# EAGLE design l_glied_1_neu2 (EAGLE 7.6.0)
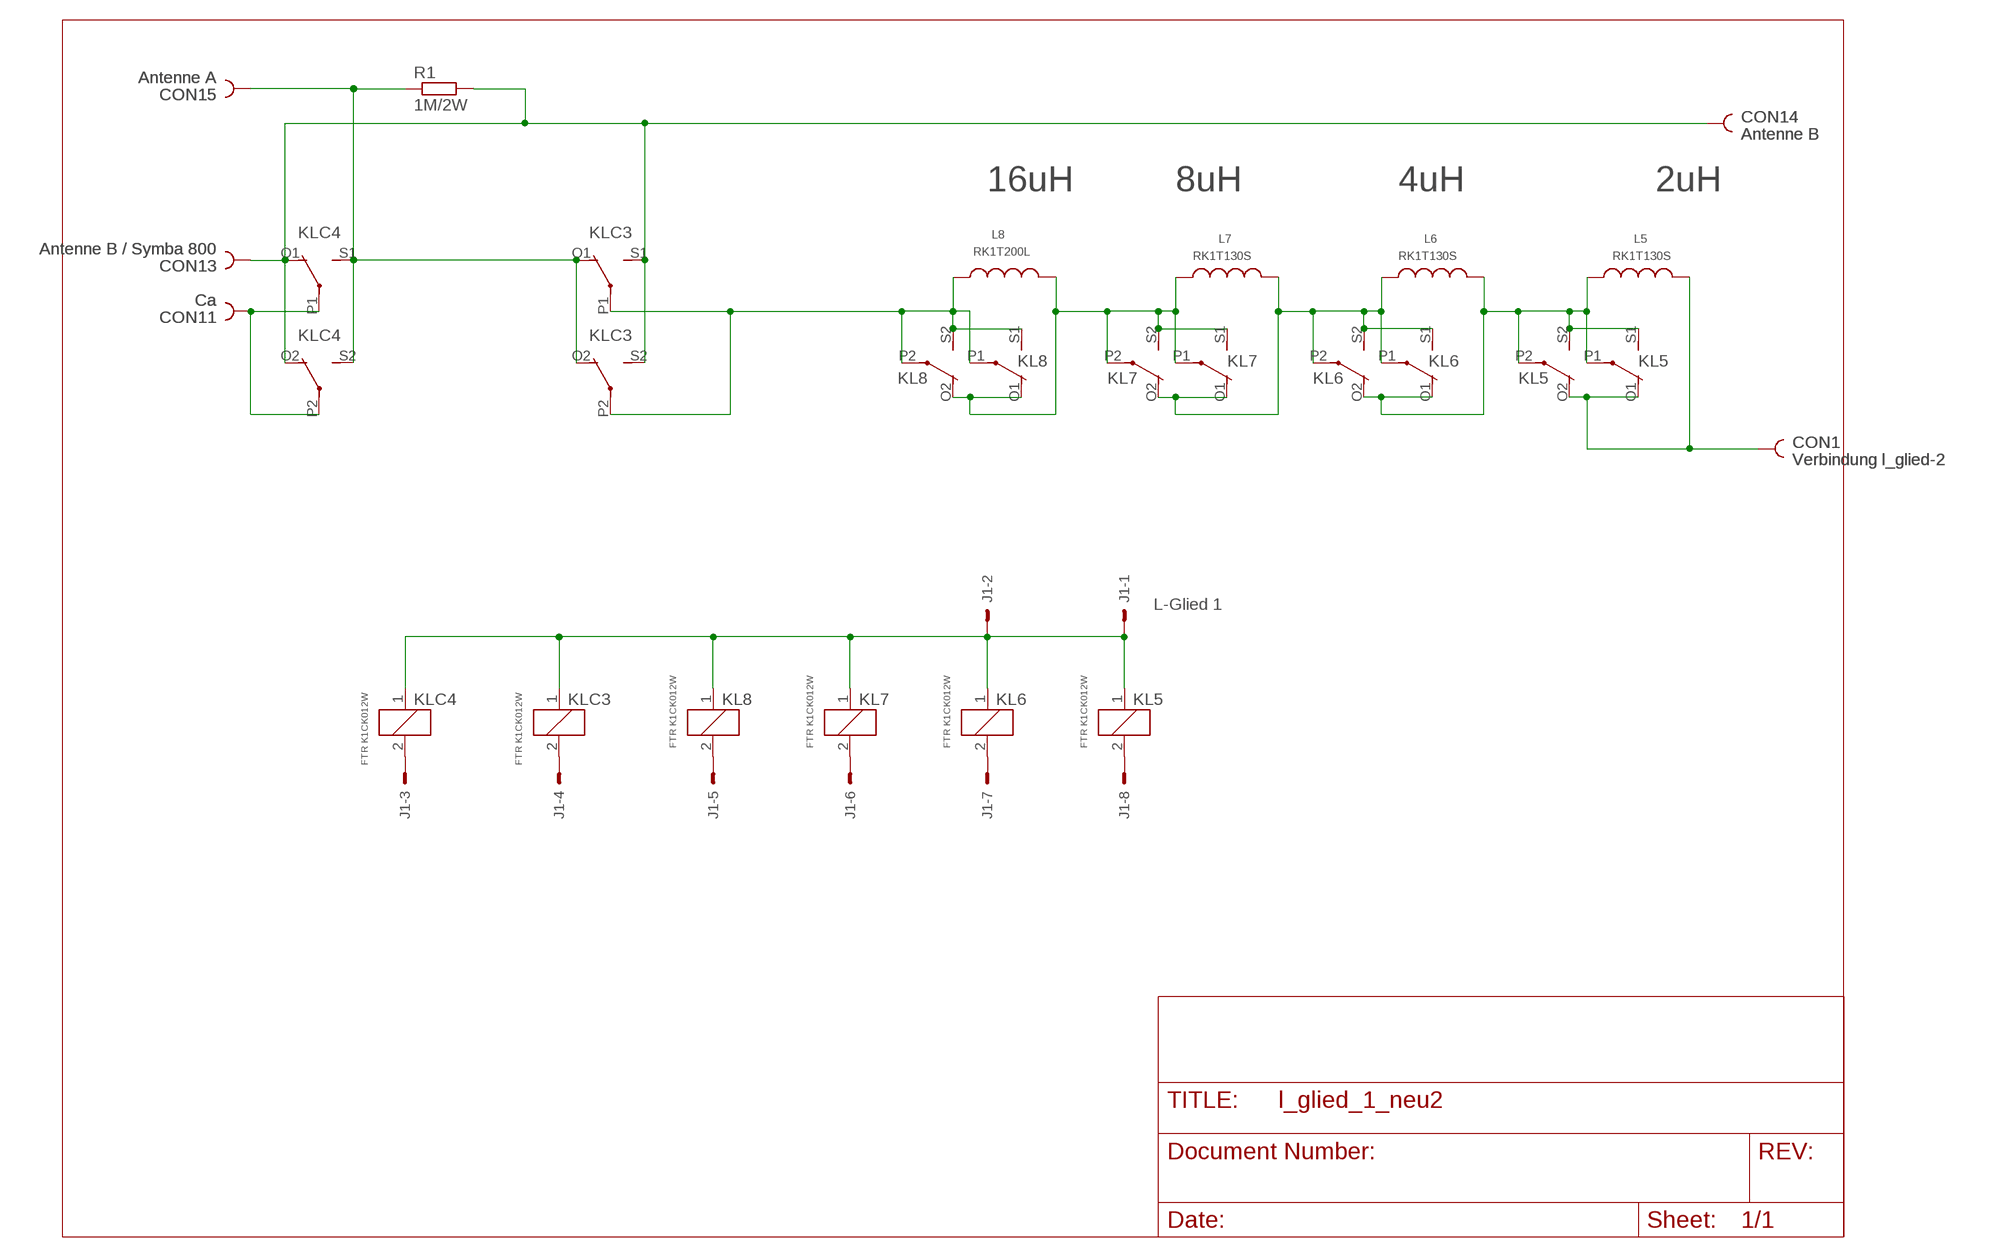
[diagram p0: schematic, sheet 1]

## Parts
CON1  Verbindung l_glied-2  PIN2_53MM  [HOLE3]
CON11  Ca  PIN2_53MM  [HOLE3]
CON13  Antenne B / Symba 800  PIN2_53MM  [HOLE3]
CON14  Antenne B  PIN2_53MM  [HOLE3]
CON15  Antenne A  PIN2_53MM  [HOLE3]
J1  L-Glied 1  22-27-2081-08  [6410-08]
KL5  FTR K1CK012W  4052  [F4052]
KL6  FTR K1CK012W  4052  [F4052]
KL7  FTR K1CK012W  4052  [F4052]
KL8  FTR K1CK012W  4052  [F4052]
KLC3  FTR K1CK012W  4052  [F4052]
KLC4  FTR K1CK012W  4052  [F4052]
L5  RK1T130S  [T130S]
L6  RK1T130S  [T130S]
L7  RK1T130S  [T130S]
L8  RK1T200L  [T200L]
R1  1M/2W  R-EU_R2512  [R2512]

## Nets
N$1: KL7.P1(2:P) KL7.P2(3:P) KL7.S1(2:S) KL7.S2(3:S) KL8.O1(2:O) KL8.O2(3:O) L7.1 L8.2
N$2: J1.5 KL8.2
N$3: KL5.P1(2:P) KL5.P2(3:P) KL5.S1(2:S) KL5.S2(3:S) KL6.O1(2:O) KL6.O2(3:O) L5.1 L6.2
N$4: J1.6 KL7.2
N$5: J1.7 KL6.2
N$6: J1.4 KLC3.2
N$7: J1.8 KL5.2
N$8: CON13.1 CON14.1 KLC3.S1(2:S) KLC3.S2(3:S) KLC4.O1(2:O) KLC4.O2(3:O) R1.2
N$9: CON15.1 KLC3.O1(2:O) KLC3.O2(3:O) KLC4.S1(2:S) KLC4.S2(3:S) R1.1
N$11: J1.3 KLC4.2
N$15: CON11.1 KLC4.P1(2:P) KLC4.P2(3:P)
N$16: KL8.P1(2:P) KL8.P2(3:P) KL8.S1(2:S) KL8.S2(3:S) KLC3.P1(2:P) KLC3.P2(3:P) L8.1
N$18: J1.1 J1.2 KL5.1 KL6.1 KL7.1 KL8.1 KLC3.1 KLC4.1
N$37: KL6.P1(2:P) KL6.P2(3:P) KL6.S1(2:S) KL6.S2(3:S) KL7.O1(2:O) KL7.O2(3:O) L6.1 L7.2
N$39: CON1.1 KL5.O1(2:O) KL5.O2(3:O) L5.2

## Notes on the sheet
- 16uH | 8uH | 4uH | 2uH

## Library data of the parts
CON1 CON11 CON13-CON15 = lindenau:PIN2_5
J1 = con-molex:22-?-08: CONNECTOR wire to board 2.54 mm (.1 inch) pitch header; OC_FARNELL: unknown; OC_NEWARK: unknown
KL5-KL8 KLC3 KLC4 = relay:4052: RELAY 2 x switch, Finder; OC_FARNELL: unknown; OC_NEWARK: unknown
L5-L8 = lindenau:RK1
R1 = rcl:R-EU_: RESISTOR, European symbol

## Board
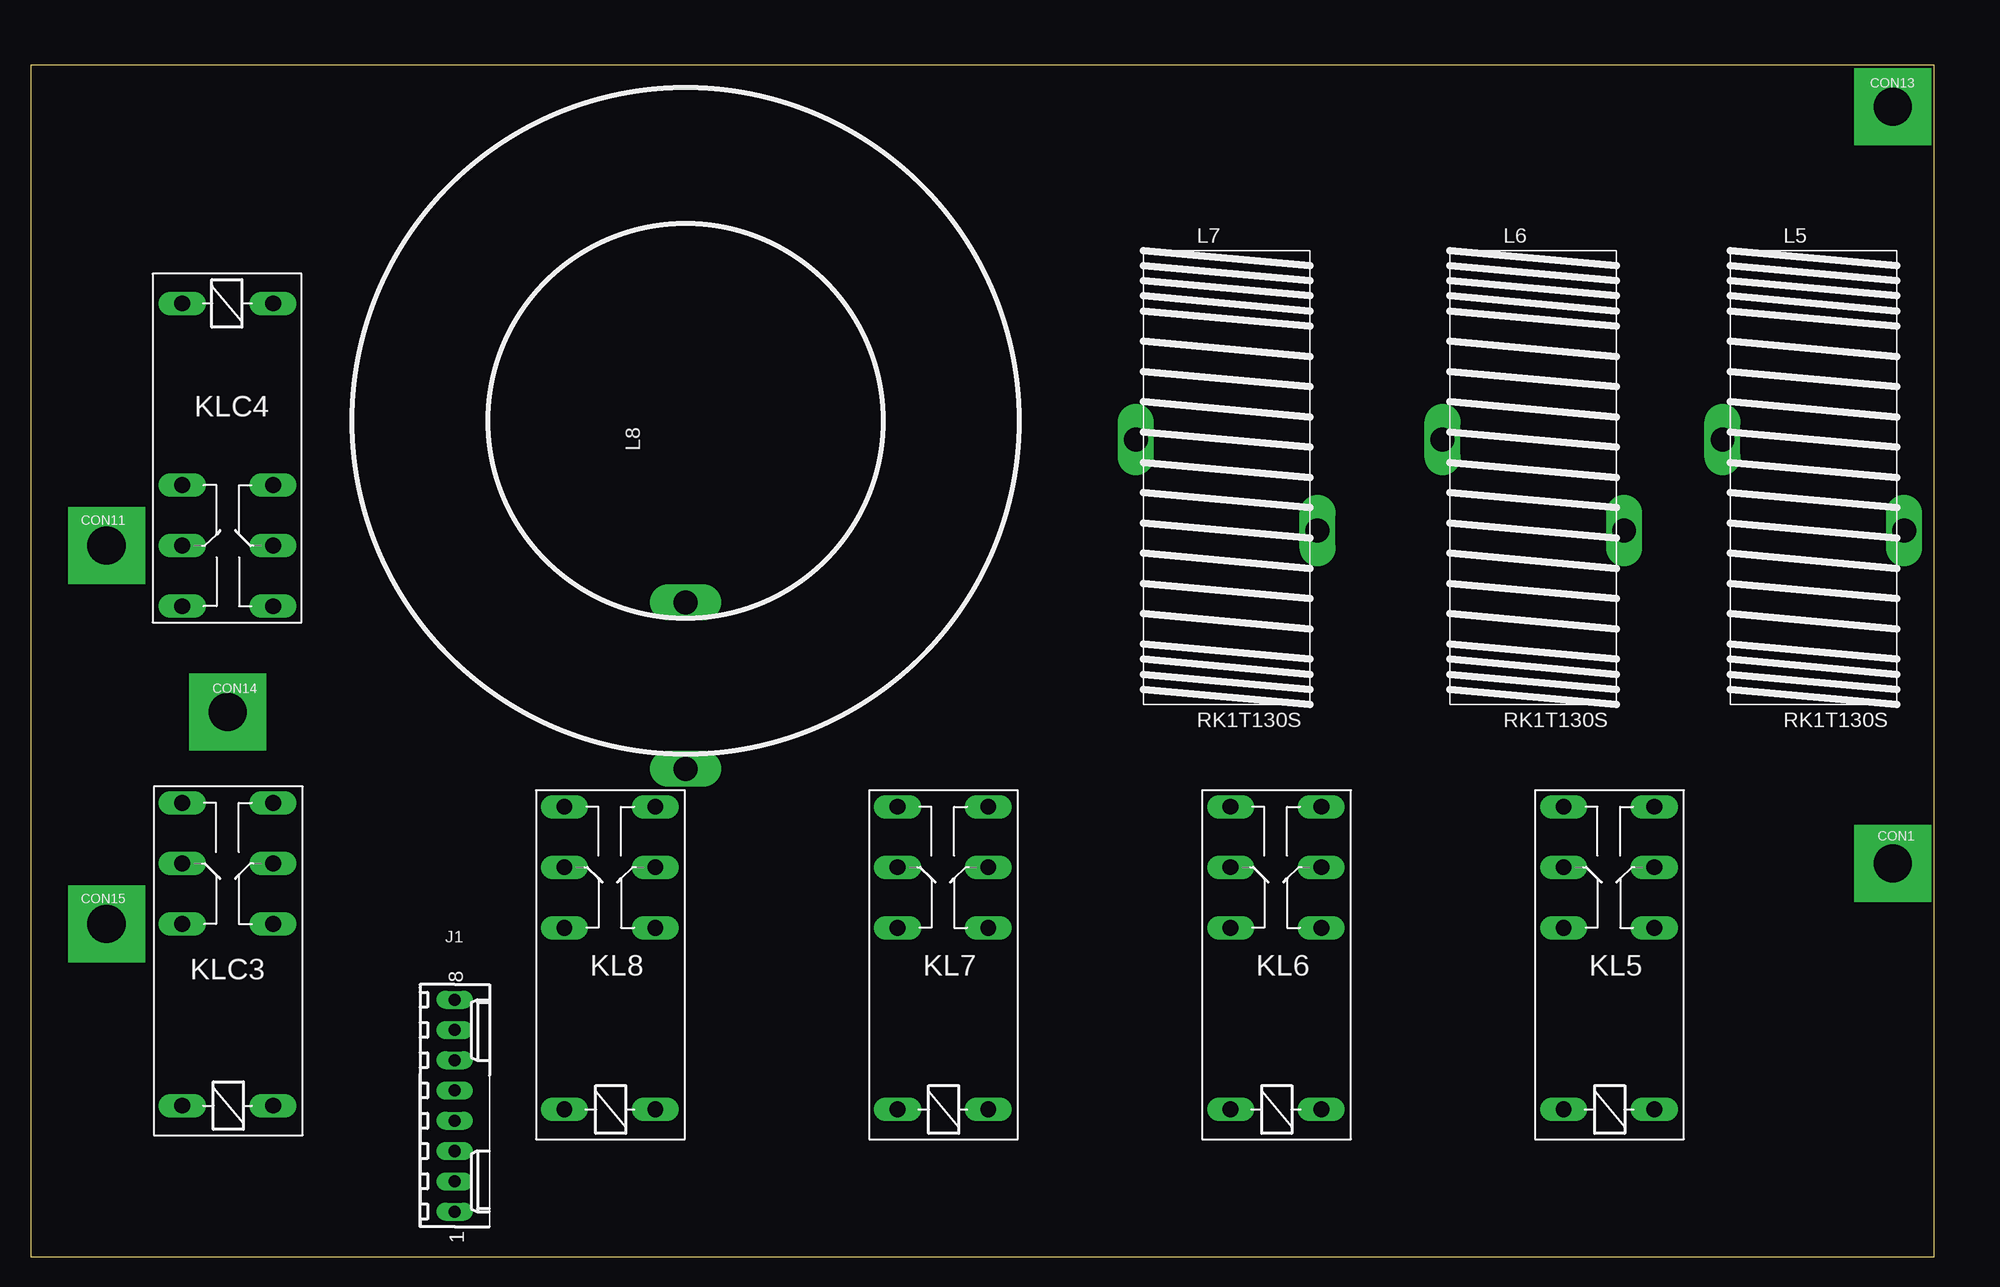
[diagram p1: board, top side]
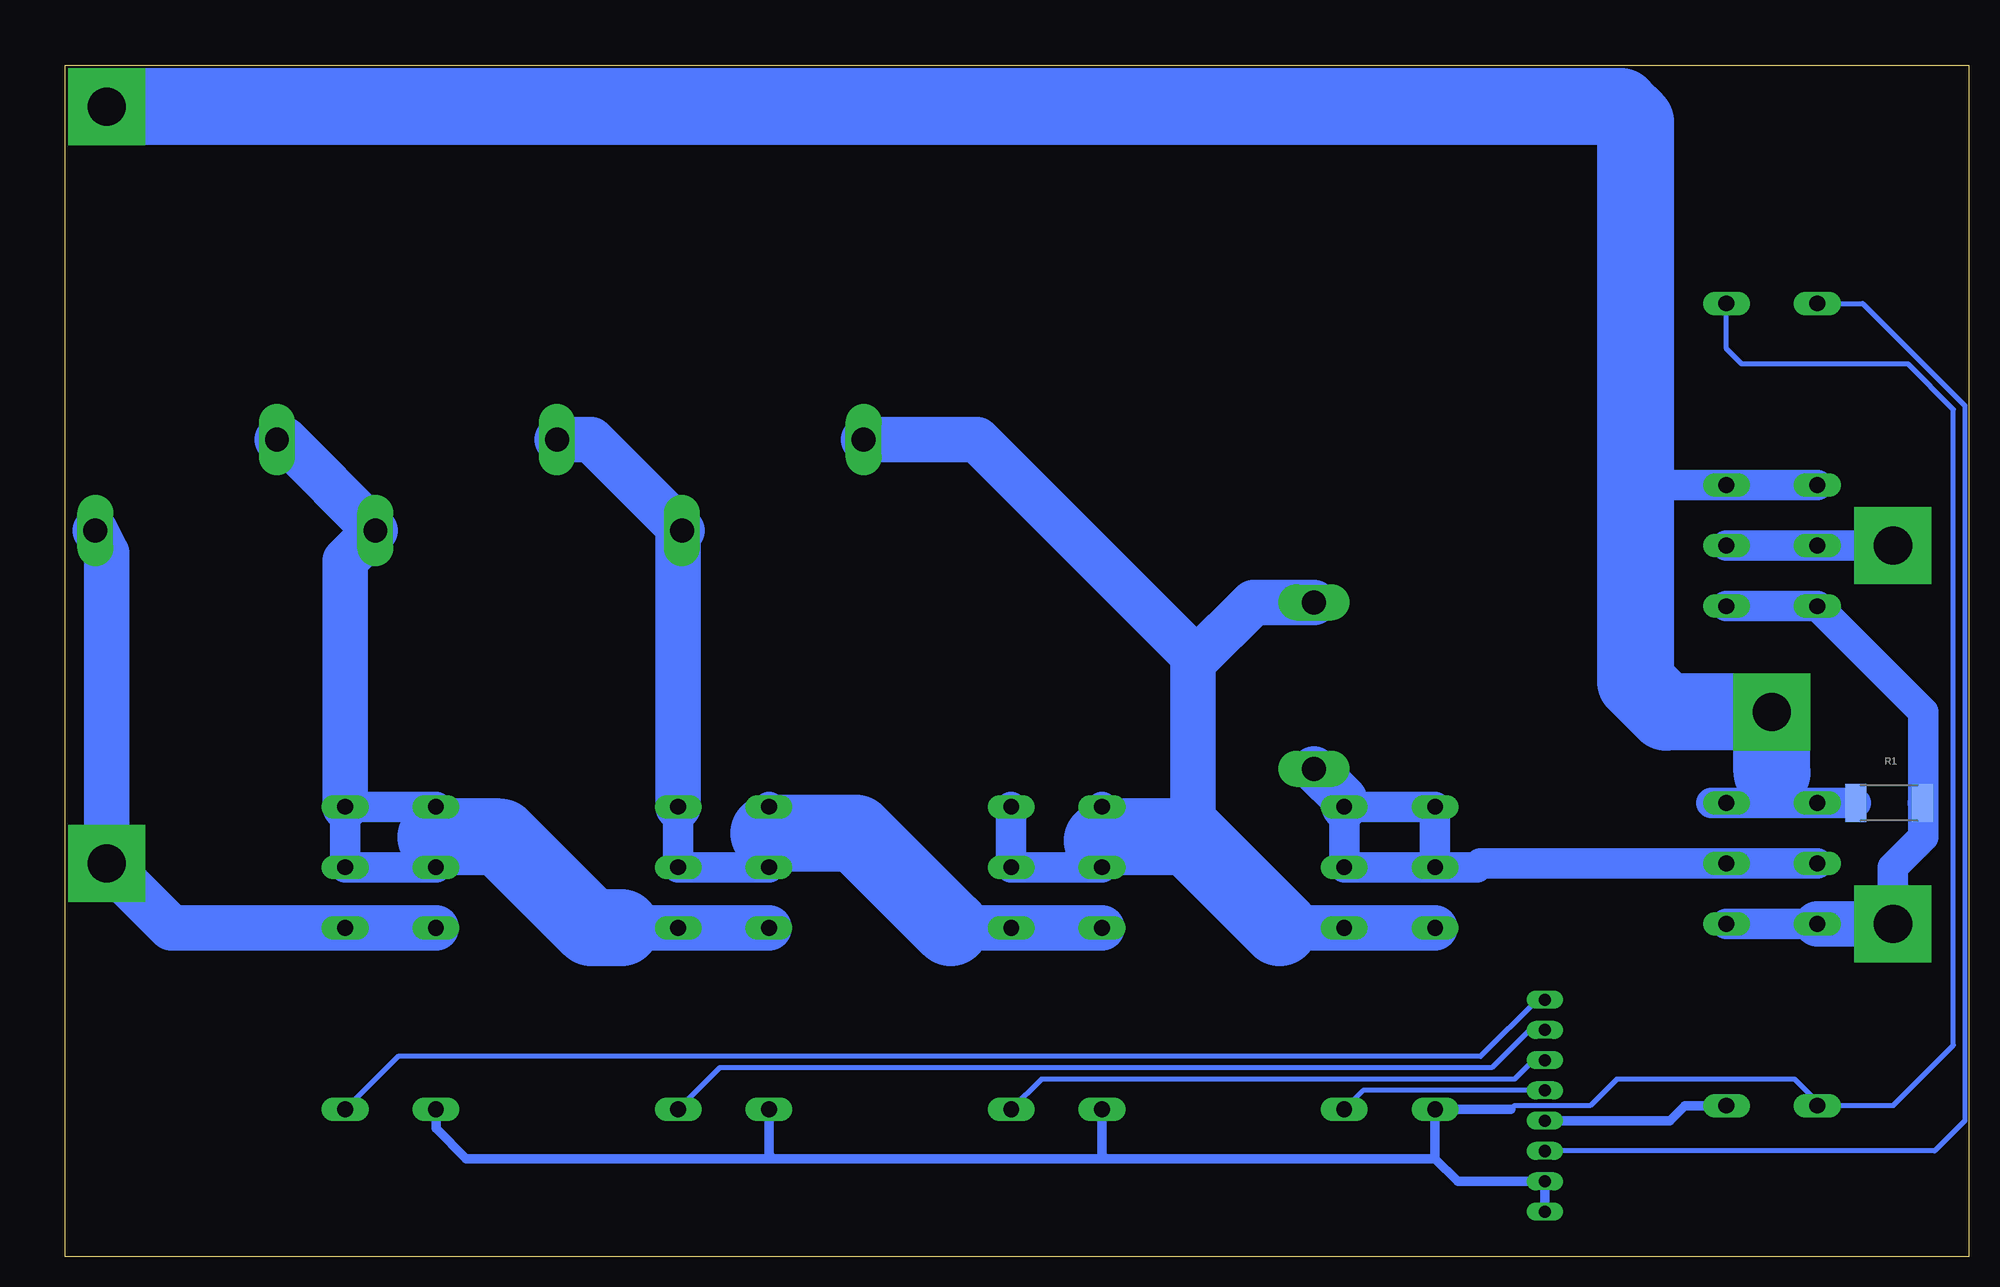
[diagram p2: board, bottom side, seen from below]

Size 159.7 x 100.01 mm. Coordinates in mm from the lower left corner, seen from the top.
Outline: 0,0 159.7,0 159.7,100.01 0,100 0,0
Copper layers (1*16): Top 0.035mm / dielectric 1.5mm / Bottom 0.035mm
Design rules "default": minimum track width 10mil, minimum drill 24mil, track to track 8mil, track to pad 8mil, pad to pad 8mil, via to via 8mil, smd to smd 8mil, copper to edge 40mil, drill to drill 8mil, minimum pad ring 10mil, minimum via ring 8mil, stop-mask expansion 4mil, vias tented up to drill 0mil, thermal gap 10mil

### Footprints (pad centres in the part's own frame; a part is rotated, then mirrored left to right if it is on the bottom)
HOLE3 = drill 3.2 pad 6.452 square: 1 0,0
6410-08 = drill 1.016 long: 1 8.89,0; 2 6.35,0; 3 3.81,0; 4 1.27,0; 5 -1.27,0; 6 -3.81,0; 7 -6.35,0; 8 -8.89,0
F4052 = drill 1.321 long: 1 -3.81,3.81; 2 -3.81,-3.81; O1 11.43,-3.81; O2 11.43,3.81; P1 16.51,-3.81; P2 16.51,3.81; S1 21.59,-3.81; S2 21.59,3.81
T130S = drill 2 long: 1 -7.62,3.81; 2 7.62,-3.81
T200L = drill 2 long: 1 -29.21,0; 2 -15.24,0
R2512 = smd 1.8 x 3.2: 1 -2.8,0; 2 2.8,0

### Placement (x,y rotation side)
CON1  156.21,33.02 0 top
CON11  6.35,59.69 0 top
CON13  156.21,96.52 0 top
CON14  16.51,45.72 0 top
CON15  6.35,27.94 0 top
J1  35.56,12.7 270 top
KL5  132.4,16.19 90 top
KL6  104.46,16.19 90 top
KL7  76.52,16.19 90 top
KL8  48.58,16.19 90 top
KLC3  16.51,16.51 90 top
KLC4  16.51,76.2 270 top
L5  149.54,64.77 0 top
L6  126.05,64.77 0 top
L7  100.33,64.77 0 top
L8  54.93,70.17 90 top
R1  6.67,38.1 180 bottom

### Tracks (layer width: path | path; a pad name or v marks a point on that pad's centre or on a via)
N$1
  Bottom 2.54: KL7.S1 KL7.P1 KL7.P2 72.71,34.92 KL7.S2
  Bottom 3.81: KL8.O2 KL8.O1 57.78,27.62 | L8.2 60.01,54.93 64.77,50.16 | 64.77,50.16 65.09,49.85 65.09,36.2 65.41,35.88 65.72,35.88 66.36,35.24 | L7.1 83.19,68.58 64.77,50.16
  Bottom 6.452: 57.78,27.62 65.41,35.24 66.36,35.24 72.39,35.24 72.71,34.92
N$2
  Bottom 0.406: J1.5 50.8,13.97 KL8.2
N$3
  Bottom 2.54: KL5.P2 128.59,35.24 KL5.S2 KL5.S1 KL5.P1 KL5.P2
  Bottom 3.81: KL6.O2 KL6.O1 113.03,27.62 | L5.1 141.29,68.58 L6.2 136.21,58.42 KL5.S1
  Bottom 6.452: 113.03,27.62 115.57,27.62 123.19,35.24 128.59,35.24
N$4
  Bottom 0.406: J1.6 36.51,16.51 38.1,14.92 77.79,14.92 KL7.2
N$5
  Bottom 0.406: J1.7 36.83,19.05 40.01,15.88 104.78,15.88 KL6.2
N$6
  Bottom 0.813: KLC3.2 23.81,12.7 25.08,11.43 J1.4
N$7
  Bottom 0.406: J1.8 36.2,21.59 40.96,16.83 131.76,16.83 KL5.2
N$8
  Bottom 2.54: 16.51,38.1 KLC3.S2 R1.2 | 16.51,38.1 KLC3.S1 21.59,38.1 | KLC4.O1 KLC4.O2 27.94,64.77 | 16.51,38.1 16.51,40.64
  Bottom 6.452: 16.51,40.64 CON14.1 25.4,45.72 27.94,48.26 27.94,64.77 27.94,95.25 29.21,96.52 CON13.1
N$9
  Bottom 2.54: KLC3.O2 KLC3.O1 | KLC4.S2 KLC4.S1 3.81,45.72 3.81,38.16 R1.1 3.81,38.04 3.81,35.24 6.35,32.7 CON15.1
  Bottom 3.81: CON15.1 KLC3.O2
N$11
  Bottom 0.406: KLC4.2 8.89,80.01 0.32,71.44 0.32,11.43 2.86,8.89 J1.3
N$15
  Bottom 2.54: CON11.1 KLC4.P1 KLC4.P2
N$16
  Bottom 2.54: KLC3.P2 KLC3.P1 40.96,33.02 41.27,32.7 KL8.P2 | KL8.P2 KL8.P1 KL8.S1 KL8.S2 KL8.P2
  Bottom 3.81: KL8.S1 52.39,38.42 L8.1
N$18
  Bottom 0.406: KLC4.1 20.32,76.2 19.05,74.93 5.08,74.93 1.27,71.12 1.27,17.78 6.35,12.7 KLC3.1 12.7,13.02 14.61,14.92 29.53,14.92 31.75,12.7 38.1,12.7 38.42,12.38
  Bottom 0.813: 38.42,12.38 KL8.1 44.77,8.26 | J1.1 J1.2 42.86,6.35 44.77,8.26 | 44.77,8.26 72.39,8.26 | 72.39,8.26 100.33,8.26 | 100.33,8.26 126.05,8.26 128.59,10.79 KL5.1 | KL6.1 100.65,8.57 100.33,8.26 | KL7.1 72.71,8.57 72.39,8.26
N$37
  Bottom 2.54: KL6.S1 KL6.P1 KL6.P2 100.65,35.56 KL6.S2
  Bottom 3.81: KL7.O2 KL7.O1 85.41,27.62 | L6.1 115.57,68.58 L7.2 108.27,60.64 KL6.S1
  Bottom 6.452: 85.41,27.62 93.34,35.56 100.65,35.56
N$39
  Bottom 3.81: KL5.O2 KL5.O1 150.81,27.62 CON1.1 156.21,59.05 L5.2

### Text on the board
Document: Relais KL5 | Relais KL6 | Relais KL7 | Relais KL8 | Relais KLC3 | Relais KLC4 | 12 Volt | 12 Volt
